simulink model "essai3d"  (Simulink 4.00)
settings: Solver=ode45  SolverMode=SingleTasking  StartTime=0.0  StopTime=tend  FixedStep=[]  MaxStep=1  RelTol=1e-3  AbsTol=1e-3
PreLoadFcn:
  | demo2dat
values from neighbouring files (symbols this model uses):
  delt = 0.2    [demo1dat.m]    (also in essai1dat.m; essai2dat.m = 0.1)
  m = 4    [demo1dat.m]    (also in demo2dat.m = 3; essai1dat.m; essai2dat.m = 6; mynlcmpc.m = mp(1:max(size(mp))-1))
  model = tfd2step(1.6,delt,1,g)    [essai2dat.m]    (also in mynlcmpc.m = modelpd(:,1:nu); mynlcmpc2.m = modelpd(:,1:nu); mynlcmpc3.m = modelpd(:,1:nu); scrtp1.m = tfd2step(tfinal,Ts,1,g))
  p = 10    [demo1dat.m]    (also in demo2dat.m; essai1dat.m; essai2dat.m; mynlcmpc.m = mp(max(size(mp))))
  r = [68.3 2]    [demo1dat.m]    (also in demo2dat.m = [0 0 0]; essai1dat.m; essai2dat.m = 10; mynlcmpc.m = zeros(1,ny))
  ulim = [-5 40 3]    [essai2dat.m]    (also in mynlcmpc.m = [-inf*ones(1,nu) inf*ones(1,nu) 1e6*ones(1,nu)]; mynlcmpc2.m = [-inf*ones(1,nu) inf*ones(1,nu) 1e6*ones(1,nu)]; mynlcmpc3.m = [-inf*ones(1,nu) inf*ones(1,nu) 1e6*ones(1,nu)]; pmlin.m = [-10*[1 1] 10*[1 1] 2*[1 1]])
  uwt = [0 0]    [demo1dat.m]    (also in demo2dat.m = 0.6*[1 1]; essai1dat.m; essai2dat.m = 1; mynlcmpc.m = ryuwt(:,2*ny+1:2*ny+nu))
  ylim = [-40 40]    [essai2dat.m]    (also in mynlcmpc.m = [ylim; ylim(N,:)]; mynlcmpc2.m = [ylim; ylim(N,:)]; mynlcmpc3.m = [ylim; ylim(N,:)]; pmlin.m = [])
  ywt = [1 1]    [demo1dat.m]    (also in demo2dat.m = [0.2,0,1]; essai1dat.m; essai2dat.m = 1; mynlcmpc.m = ryuwt(:,ny+1:2*ny))

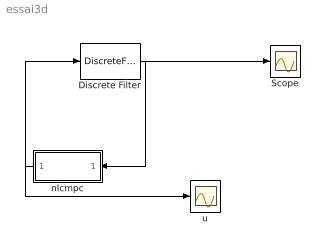
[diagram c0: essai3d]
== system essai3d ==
  Discrete Filter : DiscreteFilter  Numerator="[ 0  0  1]"  Denominator=[1 0.5]  SampleTime=delt  Realization=auto
  Scope : Scope
  nlcmpc : Subsystem  Orientation=left  AncestorBlock=nlmpclib/nlcmpc  mask(myCMPC-SIMULINK){modelpd=[model []], ryuwt=[r ywt uwt], mp=[m p], yulim=[ylim ulim], tfilter=[], ud0=[0 []']}
      mask help: Masked MATLAB function block calls nlcmpc, links CMPC and SIMULINK.
  u : Scope
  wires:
  nlcmpc/1(Out1) -> u/1, Discrete Filter/1
  Discrete Filter/1 -> Scope/1, nlcmpc/1(In1)

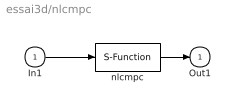
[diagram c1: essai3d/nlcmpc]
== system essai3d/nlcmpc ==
  In1 : Inport  Port=1  LatchInput=off
  nlcmpc : S-Function  FunctionName=mynlcmpc  Parameters=modelpd,mp,tfilter,ryuwt,ud0,yulim  PortCounts=[]  SFunctionModules=''
  Out1 : Outport  Port=1  InitialOutput=0
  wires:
  In1/1 -> nlcmpc/1
  nlcmpc/1 -> Out1/1
